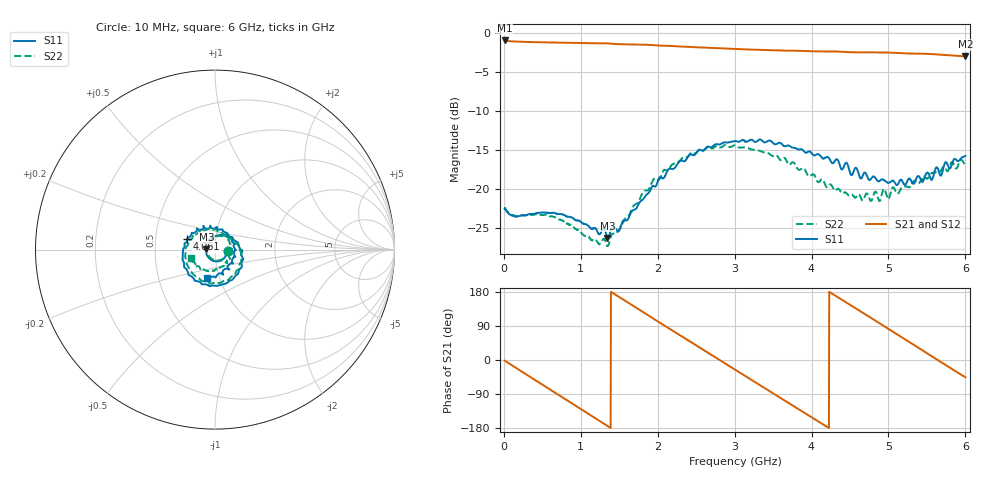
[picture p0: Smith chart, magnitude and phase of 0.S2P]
!Agilent Technologies,E5071C,MY46316741,A.11.02
!Date: Thu Jul 30 16:08:43 2020
!Data & Calibration Information:
!Freq	S11:SOLT4(ON)	S21:SOLT4(ON)	S12:SOLT4(ON)	S22:SOLT4(ON)
!PortZ  Port1:50+j0  Port2:50+j0
!Above PortZ is port z conversion or system Z0 setting when saving the data.
!When reading, reference impedance value at option line is always used.
# Hz S dB R 50
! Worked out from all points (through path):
!   1561 points, 10 MHz to 6 GHz, reference 50 ohm
!   highest |S21| = -0.94 dB at 10 MHz (marker M1); lowest = -3.0 dB at 6 GHz (marker M2)
!   group delay of S21, straight-line fit = 354 ps
!   lowest |S11| = -26.4 dB at 1.346 GHz (marker M3), VSWR 1.10, Z = 45.4 + j0.249 ohm
!   |S11| at or under -10 dB: start of sweep to end of sweep
!   |S22| runs from -27.4 to -14.4 dB; largest |S21 - S12| = 0.011
!   S11 on the Smith chart (normalised r, x): 10 MHz: 1.16, -0.01; 4.061 GHz: 0.73, +0.09; 6 GHz: 0.88, -0.28
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1e7  -22.55 -4.2  -0.94 -1.6  -0.94 -1.6  -22.48 -4.0
2.634231e8  -23.42 -20.0  -1.12 -34.5  -1.12 -34.6  -23.43 -22.3
5.475641e8  -23.07 -46.7  -1.19 -71.1  -1.18 -71.1  -23.37 -50.9
7.74109e8  -23.36 -74.8  -1.23 -100.2  -1.22 -100.3  -24.16 -80.1
1.012173e9  -24.38 -112.7  -1.27 -130.8  -1.27 -131.0  -25.76 -121.1
1.346231e9  -26.36 176.7  -1.32 -173.9  -1.31 -174.1  -27.40 157.2
1.649571e9  -23.12 101.8  -1.45 147.2  -1.45 147.0  -22.93 85.1
2.006667e9  -18.91 38.3  -1.59 101.2  -1.58 101.0  -18.89 23.3
2.26009e9  -16.79 -0.3  -1.71 68.8  -1.69 68.4  -16.55 -13.5
2.563429e9  -15.05 -36.1  -1.84 30.4  -1.83 30.0  -14.97 -54.9
2.786135e9  -14.30 -62.2  -1.93 2.2  -1.92 1.7  -14.53 -83.9
3.005e9  -13.89 -86.6  -2.01 -25.6  -2.01 -26.1  -14.43 -113.0
3.266103e9  -13.99 -115.1  -2.13 -58.5  -2.13 -58.9  -15.01 -146.3
3.504167e9  -14.16 -141.1  -2.21 -88.5  -2.19 -89.1  -15.78 -179.4
3.742231e9  -14.67 -166.4  -2.25 -118.4  -2.25 -119.0  -16.67 146.2
4.007173e9  -15.52 166.8  -2.33 -151.9  -2.31 -152.6  -18.20 109.0
4.060929e9  -15.62 158.9  -2.35 -158.7  -2.33 -159.3  -18.75 102.1
4.471782e9  -16.97 117.0  -2.44 149.0  -2.44 148.3  -20.78 36.1
4.755923e9  -18.90 79.4  -2.47 113.3  -2.47 112.5  -21.35 -4.4
5.001667e9  -19.25 41.1  -2.50 81.7  -2.50 80.9  -21.36 -36.6
5.516192e9  -17.98 -36.6  -2.67 15.9  -2.66 15.1  -18.62 -99.3
6e9  -15.77 -105.1  -2.99 -45.7  -2.97 -46.6  -16.94 -159.7
